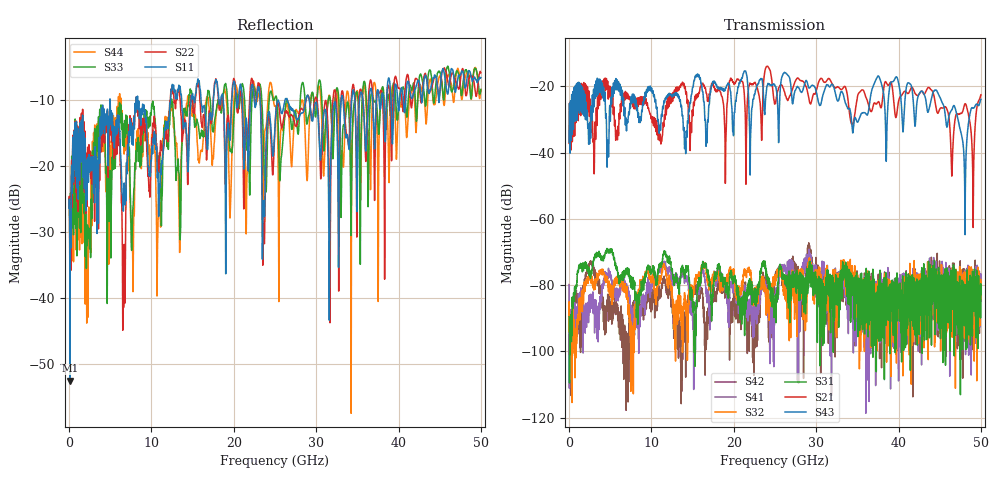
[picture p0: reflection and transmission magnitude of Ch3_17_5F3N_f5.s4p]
!Agilent Technologies,N5247A,US51170199,A.09.90.13
!Agilent N5247A: A.09.90.13
!Date: Wednesday, December 09, 2015 09:29:30
!Correction: S11(Full 4 Port(1,2,3,4))
!S12(Full 4 Port(1,2,3,4))
!S13(Full 4 Port(1,2,3,4))
!S14(Full 4 Port(1,2,3,4))
!S21(Full 4 Port(1,2,3,4))
!S22(Full 4 Port(1,2,3,4))
!S23(Full 4 Port(1,2,3,4))
!S24(Full 4 Port(1,2,3,4))
!S31(Full 4 Port(1,2,3,4))
!S32(Full 4 Port(1,2,3,4))
!S33(Full 4 Port(1,2,3,4))
!S34(Full 4 Port(1,2,3,4))
!S41(Full 4 Port(1,2,3,4))
!S42(Full 4 Port(1,2,3,4))
!S43(Full 4 Port(1,2,3,4))
!S44(Full 4 Port(1,2,3,4))
!S4P File: Measurements: <S11,S12,S13,S14>,
!<S21,S22,S23,S24>,
!<S31,S32,S33,S34>,
!<S41,S42,S43,S44>:
# Hz S  dB  R 50
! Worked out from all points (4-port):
!   3201 points, 10 MHz to 50 GHz, reference 50 ohm
!   strongest paths, dB at 10 MHz, 12.51 GHz, 25 GHz, 37.5 GHz, 50 GHz:
!     S43: -36.9, -23.0, -19.9, -16.9, -24.0
!     S21: -37.2, -22.5, -25.2, -24.7, -22.6
!     S31: -89.5, -75.0, -87.3, -82.9, -82.8
!     S32: -91.0, -82.1, -79.4, -95.0, -78.3
!     S41: -80.0, -77.4, -85.4, -85.5, -83.4
!     S42: -79.8, -84.1, -78.4, -81.8, -84.7
!   lowest |S11| = -52.4 dB at 119.4 MHz (marker M1), VSWR 1.00, Z = 50.1 + j0.233 ohm
!   |S11| at or under -10 dB: start of sweep to 4.961 GHz; 8.346 GHz to 12.32 GHz (3.974 GHz wide, 38.5 % of centre); 29.17 GHz to 33.04 GHz (3.87 GHz wide, 12.4 % of centre)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
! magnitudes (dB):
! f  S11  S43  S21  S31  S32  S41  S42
! 10 MHz  -26.4  -36.9  -37.2  -89.5  -91.0  -80.0  -79.8
! 119.4 MHz  -52.4  -40.2  -36.2  -99.1  -103.3  -98.7  -95.1
! 24.08 GHz  -12.9  -19.7  -13.9  -78.2  -83.6  -82.0  -83.2
! 39.71 GHz  -7.7  -17.2  -29.4  -88.4  -79.4  -91.8  -96.1
! 48.05 GHz  -8.0  -53.2  -25.4  -91.9  -82.1  -75.7  -92.2
! 49.03 GHz  -6.9  -26.5  -50.6  -78.8  -84.1  -83.0  -90.0
! 50 GHz  -6.6  -24.0  -22.6  -82.8  -78.3  -83.4  -84.7
